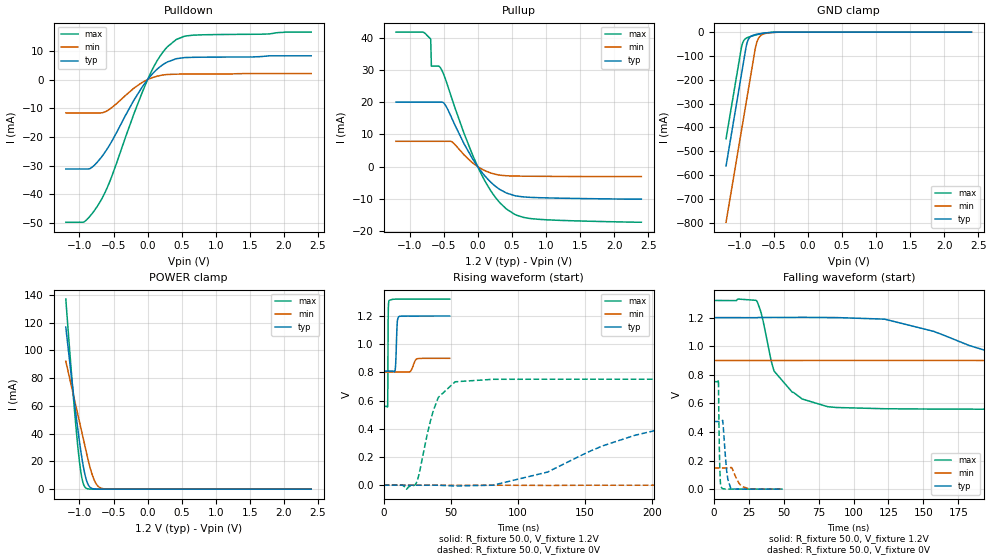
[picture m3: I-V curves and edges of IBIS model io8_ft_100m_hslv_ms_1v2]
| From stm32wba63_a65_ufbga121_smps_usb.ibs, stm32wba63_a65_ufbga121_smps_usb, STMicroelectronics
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[Model]   io8_ft_100m_hslv_ms_1v2
Model_type I/O
Polarity   Non-Inverting
Enable   Active-Low
| CAP_THRESHOLD on pad IOFT is "UDTCAPC" :
| Rising=30.0% of vddiom   Falling=70.0% of vddiom
| C_comp min and max val. don't necessarily correlate with the min and max pvt
| but are the smallest and greatest pad capacitance found.
| var   typ   min   max
C_comp   2.96003pF  2.88430pF  3.14833pF
|C_comp_pullup   1.71850pF  1.56046pF  1.93937pF
|C_comp_pulldown   1.24153pF  1.32384pF  1.20896pF
Vinl = 450.0mV
Vinh = 660.0mV
Vmeas = 600.0mV   | Reference voltage for timing measurements
Cref  = 50.0pF   | Timing specification test load capacitance value
Rref  = 1.0MOhm   | Timing specification test load resistance value
Vref  = 660.0mV   | Timing specification test load voltage
[Model Spec]
| TIME_THRESHOLD on pin ZIV11 is "CMOS" :
| Rising=50.0% of vdd   Falling=50.0% of vdd
Vinl 441.50000mV 335.50000mV 487.50000mV
Vinh 755.50000mV 552.50000mV 839.50000mV
| variable   typ   min   max
[Temperature Range] 25.0 140.0 -40.0
| variable   typ   min   max
[Voltage Range] 1.2V 900.0mV 1.32V
| variable   typ   min   max
[POWER Clamp Reference] 1.2V 900.0mV 1.32V
| variable   typ   min   max
[GND Clamp Reference] 0V 0V 0V
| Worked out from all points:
|   slope of the pulldown table from 0 to 0.18 V, typ, clamps not added: 40.6 ohm
|   slope of the pullup table from 0 to 0.18 V, typ, clamps not added: 39.4 ohm
|   GND clamp passes 1 mA (typ) near -0.51 V on its own axis
|   POWER clamp passes 1 mA (typ) near -0.83 V on its own axis
|   rising waveform, R_fixture 50.0, V_fixture 1.2V: 20-80 % time 856ps typ, 2.39ns min, 235ps max; typ from 0.809 V to 1.2 V
|   falling waveform, R_fixture 50.0, V_fixture 1.2V: 20-80 % time 85.8ns typ, 201ns min, 17.8ns max; typ from 1.2 V to 0.809 V
|   rising waveform, R_fixture 50.0, V_fixture 0V: 20-80 % time 75.7ns typ, 186ns min, 11.9ns max; typ from 0 V to 0.473 V
|   falling waveform, R_fixture 50.0, V_fixture 0V: 20-80 % time 2.48ns typ, 4.72ns min, 799ps max; typ from 0.473 V to 0 V
[POWER Clamp]
-1.2V     116.7mA    92.13mA    136.9mA
-1.09V    69.42mA    68.21mA    67.14mA
-1.02V    41.75mA    52.99mA    28.91mA
-990mV    30.98mA    46.47mA    16.09mA
-970mV    24.36mA    42.12mA    9.575mA
-940mV    15.59mA    35.6mA     3.485mA
-910mV    8.693mA    29.07mA    1.01mA
-860mV    2.259mA    18.59mA    104.6uA
-780mV    143.1uA    6.246mA    2.554uA
-720mV    16.22uA    1.846mA    157.1nA
-650mV    1.267uA    330.3uA    6.114nA
2.4V      0A         0A         0A
[GND Clamp]
-1.2V     -561.6mA   -797.4mA   -447.4mA
-980mV    -187.6mA   -423.4mA   -73.43mA
-960mV    -153.6mA   -389.4mA   -48.26mA
-900mV    -54.17mA   -287.4mA   -24.97mA
-870mV    -29.55mA   -236.4mA   -21.19mA
-830mV    -17.05mA   -168.4mA   -17.42mA
-760mV    -9.921mA   -54.55mA   -11.89mA
-730mV    -8.191mA   -29.78mA   -9.811mA
-690mV    -6.26mA    -14.49mA   -7.318mA
-600mV    -2.976mA   -4.315mA   -3.058mA
-380mV    -57.63uA   -251uA     -19.49uA
2.4V      871.4pA    205.6nA    347.3pA
| variable   typ   min   max
[Pullup Reference] 1.2V 900.0mV 1.32V
| variable   typ   min   max
[Pulldown Reference] 0V 0V 0V
[Pullup]
-1.2V     20mA       7.861mA    41.7mA
-800mV    20mA       7.861mA    41.67mA
-690mV    20mA       7.861mA    39.54mA
-680mV    20mA       7.861mA    31.16mA
-530mV    20mA       7.861mA    30.04mA
-470mV    18.9mA     7.861mA    26.89mA
-370mV    14.54mA    7.569mA    20.52mA
10mV      -297.9uA   -132.1uA   -454.3uA
210mV     -5.173mA   -2.076mA   -8.052mA
420mV     -8.157mA   -2.82mA    -13.11mA
790mV     -9.528mA   -2.972mA   -16.12mA
2.4V      -10.04mA   -3.075mA   -17.21mA
[Pulldown]
-1.2V     -31.2mA    -11.62mA   -49.78mA
-930mV    -31.2mA    -11.62mA   -49.64mA
-830mV    -30.86mA   -11.62mA   -47.25mA
-710mV    -28.04mA   -11.62mA   -43.19mA
-550mV    -22.55mA   -10.2mA    -35.3mA
-200mV    -7.146mA   -2.964mA   -11.89mA
40mV      1.171mA    405.8uA    2.092mA
130mV     3.416mA    1.118mA    6.182mA
230mV     5.302mA    1.613mA    9.763mA
420mV     7.288mA    1.898mA    13.99mA
670mV     7.779mA    1.924mA    15.51mA
2.4V      8.3mA      2.094mA    16.59mA
[Ramp]
dV/dt_r 283.78422mV/15.03686ns 88.90908mV/37.01512ns 450.99581mV/2.3533ns
dV/dt_f 234.65979mV/16.43915ns 57.89272mV/39.84113ns 456.73567mV/2.8104ns
R_load = 50.0
| Removed startup time: 0s 0s 0s  .
| Removed end time: 49.25ns.
[Rising Waveform]
R_fixture   = 50.0
V_fixture   = 1.2V
V_fixture_min = 900.0mV
V_fixture_max = 1.32V
0s        808.9mV    803.5mV    558.8mV
2.95ns    808.9mV    803.5mV    561.8mV
3.1ns     808.9mV    803.5mV    662.1mV
3.3ns     808.9mV    803.5mV    1.086V
3.4ns     808.9mV    803.5mV    1.202V
4ns       808.9mV    803.5mV    1.31V
8.6ns     816.8mV    803.5mV    1.319V
10.1ns    1.148V     803.5mV    1.32V
11.05ns   1.194V     803.5mV    1.32V
49.25ns   1.2V       899.8mV    1.32V
| Removed startup time: 0s 0s 0s  .
| Removed end time: 1.99625us.
[Falling Waveform]
R_fixture   = 50.0
V_fixture   = 1.2V
V_fixture_min = 900.0mV
V_fixture_max = 1.32V
0s        1.2V       900mV      1.32V
30.5ns    1.2V       900mV      1.319V
43.25ns   1.202V     900mV      824.9mV
63.25ns   1.202V     900.2mV    630.7mV
88ns      1.2V       900.7mV    571.2mV
122.2ns   1.189V     900.4mV    562.6mV
221ns     907.1mV    900mV      559.1mV
366.8ns   818.7mV    884.3mV    558.8mV
733.5ns   808.9mV    810.1mV    558.8mV
1.996us   808.9mV    803.5mV    558.8mV
| Removed startup time: 0s 0s 0s  .
| Removed end time: 1.996us.
[Rising Waveform]
R_fixture   = 50.0
V_fixture   = 0V
V_fixture_min = 0V
V_fixture_max = 0V
0s        4.601nV    216.1nV    2.108nV
24ns      1.448uV    1.102uV    10.71mV
35.5ns    45.41uV    924.2nV    477.8mV
40.75ns   -269.6uV   923.2nV    622.9mV
53.25ns   -6.025mV   547.8nV    733.3mV
81.5ns    62.96uV    24.32uV    751.1mV
187ns     353.3mV    -11.55uV   751.6mV
285.3ns   460.4mV    8.483mV    751.6mV
651.8ns   472.8mV    140.2mV    751.6mV
1.996us   473mV      148.2mV    751.7mV
| Removed startup time: 0s 0s 0s  .
| Removed end time: 49.25ns.
[Falling Waveform]
R_fixture   = 50.0
V_fixture   = 0V
V_fixture_min = 0V
V_fixture_max = 0V
0s        473mV      148.3mV    751.7mV
3.3ns     473mV      148.3mV    764.7mV
4.1ns     473mV      148.3mV    231.7mV
4.6ns     473mV      148.3mV    73.98mV
5.05ns    473mV      148.3mV    18.02mV
6.4ns     478.3mV    148.3mV    3.512mV
9.3ns     121.7mV    148.3mV    429.3uV
12.5ns    4.309mV    152.1mV    231.1uV
21.15ns   433.8uV    15.44mV    1.734uV
49.25ns   62.93uV    101.5uV    85.22nV
